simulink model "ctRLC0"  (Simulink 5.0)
settings: Solver=ode45  StartTime=0.0  StopTime=40  MaxStep=.5  RelTol=1e-3

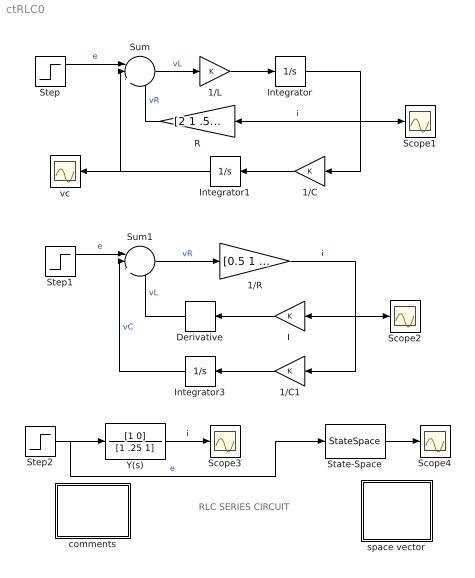
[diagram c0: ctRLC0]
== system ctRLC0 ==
  note: RLC SERIES CIRCUIT
  1/C : Gain  Orientation=left
  1/C1 : Gain  Orientation=left
  1/L : Gain
  1/R : Gain  Gain=[0.5 1 2 4]
  Derivative : Derivative  Orientation=left
  Integrator : Integrator
  Integrator1 : Integrator  Orientation=left
  Integrator3 : Integrator  Orientation=left
  L : Gain  Orientation=left
  R : Gain  Orientation=left  Gain=[2 1 .5 .25]
  Scope{1..4} (4 alike) : Scope
  State-Space : StateSpace  A=[-0.25 -1;1 0]  B=[1;0]  C=[1 0]  D=0
  Step : Step  SampleTime=0
  Step1 : Step  SampleTime=0
  Step2 : Step  SampleTime=0
  Sum : Sum  Inputs=||+--
  Sum1 : Sum  Inputs=||+--
  Y(s) : TransferFcn  Numerator=[1 0]  Denominator=[1 .25 1]
  comments : Subsystem
  space vector : Subsystem
  vc : Scope
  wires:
  Sum/1 -> 1/L/1  "vL"
  1/L/1 -> Integrator/1
  R/1 -> Sum/3  "vR"
  Step1/1 -> Sum1/1  "e"
  Sum1/1 -> 1/R/1  "vR"
  1/C/1 -> Integrator1/1
  L/1 -> Derivative/1
  1/C1/1 -> Integrator3/1
  Derivative/1 -> Sum1/3  "vL"
  1/R/1 -> L/1, 1/C1/1, Scope2/1  "i"
  Y(s)/1 -> Scope3/1  "i"
  Step2/1 -> Y(s)/1, State-Space/1  "e"
  State-Space/1 -> Scope4/1
  Integrator3/1 -> Sum1/2  "vC"
  Integrator1/1 -> Sum/2, vc/1
  Step/1 -> Sum/1  "e"
  Integrator/1 -> R/1, 1/C/1, Scope1/1  "i"

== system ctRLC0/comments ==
  note: Transient response of an RLC series circuit
  note: This demonstration illustrates different SIMULINK implementations of the transient response of an RLC series circuit: a) A feedback system representation utilizing two integrators. This arrangement is the preferred one when parametric responses are desired (such as shown by expressing the resistance R as a vector); another advantage is the inherent capability of including initial conditions. b) A feedback system representation utilizing one integrator and one differentiator. This arrangement is not recommended because of its lack of accuracy due to the presence of an algebraic loop. c) Transfer function and state-space representations are useful only when the parameters are fixed. d) Double clicking the SCRIPT block runs an ODE m-file.

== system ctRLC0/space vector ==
